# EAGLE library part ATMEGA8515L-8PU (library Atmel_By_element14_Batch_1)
Microcontroller
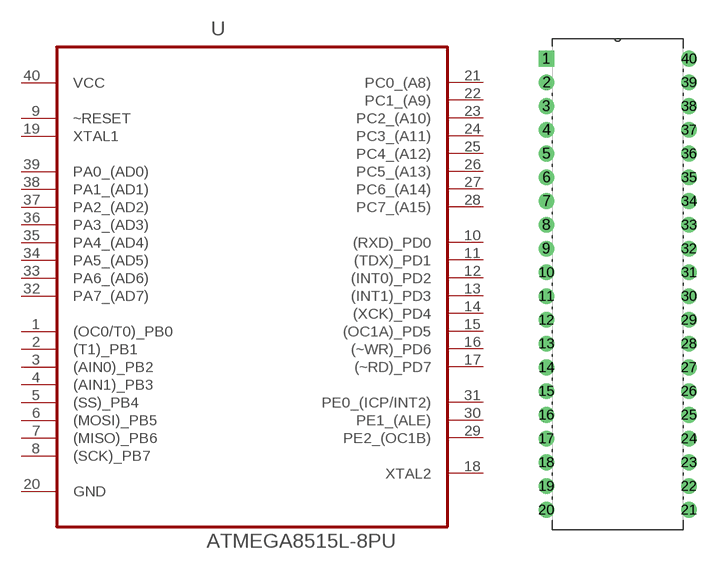
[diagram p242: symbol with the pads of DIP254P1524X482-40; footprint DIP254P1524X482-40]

Designator prefix U

## ATMEGA8515L-8PU (DESCRIPTION: Microcontroller; MPN: ATMEGA8515L-8PU; OC_FARNELL: 9171428; OC_NEWARK: 01M6907; PACKAGE: DIP-40; SUPPLIER: ATMEL)  [DIP254P1524X482-40]
1  (OC0/T0)_PB0
2  (T1)_PB1
3  (AIN0)_PB2
4  (AIN1)_PB3
5  (SS)_PB4
6  (MOSI)_PB5
7  (MISO)_PB6
8  (SCK)_PB7
9  ~RESET  in
10  (RXD)_PD0
11  (TDX)_PD1
12  (INT0)_PD2
13  (INT1)_PD3
14  (XCK)_PD4
15  (OC1A)_PD5
16  (~WR)_PD6
17  (~RD)_PD7
18  XTAL2  out
19  XTAL1  in
20  GND  pas
21  PC0_(A8)
22  PC1_(A9)
23  PC2_(A10)
24  PC3_(A11)
25  PC4_(A12)
26  PC5_(A13)
27  PC6_(A14)
28  PC7_(A15)
29  PE2_(OC1B)
30  PE1_(ALE)
31  PE0_(ICP/INT2)
32  PA7_(AD7)
33  PA6_(AD6)
34  PA5_(AD5)
35  PA4_(AD4)
36  PA3_(AD3)
37  PA2_(AD2)
38  PA1_(AD1)
39  PA0_(AD0)
40  VCC  pwr

## Footprint DIP254P1524X482-40 (pad centres in mm)
drill 1.118 square: 1 -15.24,48.26
drill 1.118: 2 -15.24,45.72; 3 -15.24,43.18; 4 -15.24,40.64; 5 -15.24,38.1; 6 -15.24,35.56; 7 -15.24,33.02; 8 -15.24,30.48; 9 -15.24,27.94; 10 -15.24,25.4; 11 -15.24,22.86; 12 -15.24,20.32; 13 -15.24,17.78; 14 -15.24,15.24; 15 -15.24,12.7; 16 -15.24,10.16; 17 -15.24,7.62; 18 -15.24,5.08; 19 -15.24,2.54; 20 -15.24,0; 21 0,0; 22 0,2.54; 23 0,5.08; 24 0,7.62; 25 0,10.16; 26 0,12.7; 27 0,15.24; 28 0,17.78; 29 0,20.32; 30 0,22.86; 31 0,25.4; 32 0,27.94; 33 0,30.48; 34 0,33.02; 35 0,35.56; 36 0,38.1; 37 0,40.64; 38 0,43.18; 39 0,45.72; 40 0,48.26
